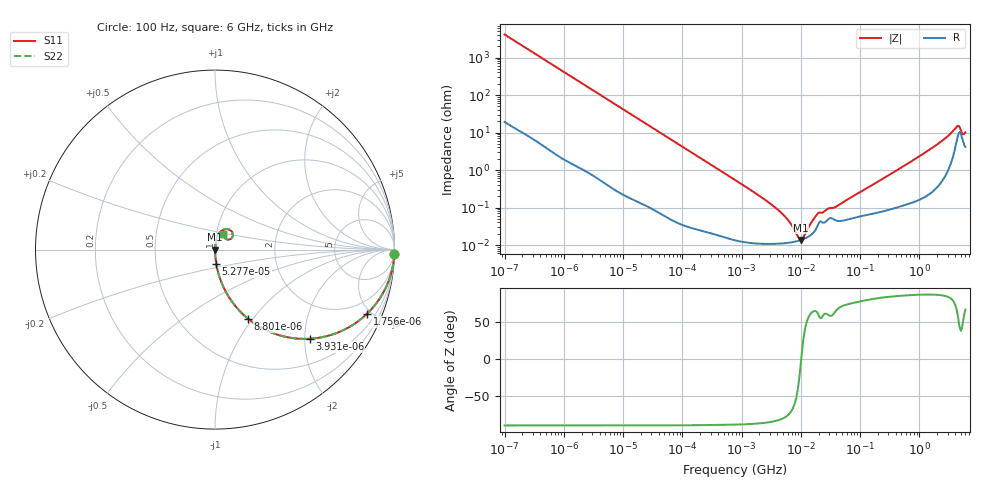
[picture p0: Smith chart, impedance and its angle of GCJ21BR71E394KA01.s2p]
!Murata Part Number: GCJ21BR71E394KA01
!These Parameters are Measured in Series Mode Connection
!Data Generated on Mar 13, 2026
!  o--ll--o
!Port1  Port2
!  o------o
!Operation Temp=25[degC], DC Bias Voltage=0[V]
!Freq. Start=100[Hz] Stop=6[GHz] 401[Steps]
# Hz S RI R 50
!Freq.(Hz) S11(Real) S11(Imag) S21(Real) S21(Imag) S12(Real) S12(Imag) S22(Real) S22(Imag)
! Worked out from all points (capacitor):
!   401 points, 100 Hz to 6 GHz, reference 50 ohm
!   read as one part in series: C = 387 nF near 109 Hz
!   lowest |Z| = 13.7 mohm at 9.942 MHz (marker M1)
!   series resonance near 10.17 MHz, so ESL is about 630 pH
!   S11 on the Smith chart (normalised r, x): 100 Hz: 1, -82; 1.756 kHz: 1.02, -4.72; 3.931 kHz: 1.01, -2.12; 8.801 kHz: 1.00, -0.95; 52.77 kHz: 1.00, -0.16; 6 GHz: 1.08, +0.19
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100  0.9993 -0.0243  0.000704 0.0243  0.000704 0.0243  0.9993 -0.0243
501  0.985 -0.1194  0.015 0.1194  0.015 0.1194  0.985 -0.1194
1756  0.8467 -0.3578  0.1533 0.3578  0.1533 0.3578  0.8467 -0.3578
2008  0.8089 -0.3906  0.1911 0.3906  0.1911 0.3906  0.8089 -0.3906
3931  0.528 -0.4966  0.472 0.4966  0.472 0.4966  0.528 -0.4966
8801  0.1845 -0.3853  0.8155 0.3853  0.8155 0.3853  0.1845 -0.3853
16473  0.0616 -0.2376  0.9384 0.2376  0.9384 0.2376  0.0616 -0.2376
40335  0.0114 -0.1027  0.9886 0.1027  0.9886 0.1027  0.0114 -0.1027
52766  0.00684 -0.0789  0.9932 0.0789  0.9932 0.0789  0.00684 -0.0789
774597  0.000164 -0.00545  0.9998 0.00545  0.9998 0.00545  0.000164 -0.00545
4246196  0.00011 -0.000829  0.9999 0.000829  0.9999 0.000829  0.00011 -0.000829
6075234  0.000115 -0.000452  0.9999 0.000452  0.9999 0.000452  0.000115 -0.000452
9090158  0.00013 -9.46e-05  0.9999 9.46e-05  0.9999 9.46e-05  0.00013 -9.46e-05
9941735  0.000136 -1.88e-05  0.9999 1.88e-05  0.9999 1.88e-05  0.000136 -1.88e-05
1.137099e7  0.000147 9.56e-05  0.9999 -9.56e-05  0.9999 -9.56e-05  0.000147 9.56e-05
1.555665e7  0.000199 0.000383  0.9998 -0.000383  0.9998 -0.000383  0.000199 0.000383
1.946e7  0.000344 0.000611  0.9997 -0.000611  0.9997 -0.000611  0.000344 0.000611
3.983537e7  0.00045 0.000967  0.9995 -0.000967  0.9995 -0.000967  0.00045 0.000967
3.124326e8  0.000932 0.00741  0.9991 -0.00741  0.9991 -0.00741  0.000932 0.00741
1.873145e9  0.00508 0.0443  0.9949 -0.0443  0.9949 -0.0443  0.00508 0.0443
4.193612e9  0.0626 0.1147  0.9374 -0.1147  0.9374 -0.1147  0.0626 0.1147
6e9  0.0472 0.0849  0.9528 -0.0849  0.9528 -0.0849  0.0472 0.0849
